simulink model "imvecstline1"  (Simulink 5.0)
settings: Solver=ode45  StartTime=0.0  StopTime=2.5  MaxStep=5e-4  RelTol=1e-3
libraries: simulink x1

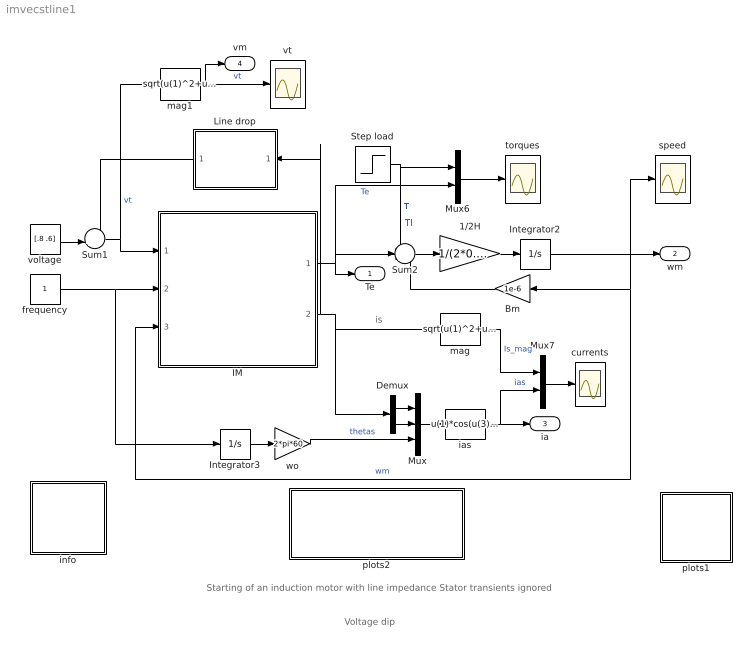
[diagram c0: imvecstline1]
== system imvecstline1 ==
  note: is
  note: Starting of an induction motor with line impedance Stator transients ignored
  note: Voltage dip
  note: Tl
  1/2H : Gain  Gain=1/(2*0.3)
  Bm : Gain  Orientation=left  Gain=1e-6
  Demux : Demux  Outputs=2
  IM : Subsystem  mask(Inductionmachine){Rs=0.01, Rr=0.02, Lsl=0.10, Lrl=0.10, Lm=4.50, wo=2*pi*60}
      mask prompts: Rs "Stator resistance [pu]"; Rr "Rotor resistance [pu]"; Lsl "Stator leakage inductance [pu]"; Lrl "Rotor leakage inductance [pu]"; Lm "Magnetizing inductance [pu]"; wo "Base frequency [rad/s]"
      mask help: Induction motor subsystem model using state space formulation in an arbitrary reference frame k. Parameters are expressed in per unit.
  Integrator2 : Integrator
  Integrator3 : Integrator
  Line drop : Subsystem  Orientation=left  mask{Rline=0.01, Lline=0.05, wo=2*pi*60}
      mask prompts: Rline "Rline [ pu]"; Lline "Lline [pu]"; wo "wo [rad/s]"
  Mux : Mux  Inputs=3
  Mux6 : Mux  Inputs=2
  Mux7 : Mux  Inputs=2
  Step load : Step  Time=2  Before=0.0  SampleTime=0
  Sum1 : Sum  Inputs=-+|
  Sum2 : Sum  Inputs=-+-
  currents : Scope
  frequency : Constant
  ias : Fcn  Expr=u(1)*cos(u(3))-u(2)*sin(u(3))
  info : Subsystem
  mag : Fcn  Expr=sqrt(u(1)^2+u(2)^2)
  mag1 : Fcn  Expr=sqrt(u(1)^2+u(2)^2)
  plots1 : Subsystem
  plots2 : Subsystem
  speed : Scope
  torques : Scope
  voltage : Constant  Value=[.8 .6]
  vt : Scope
  wo : Gain  Gain=2*pi*60
  Te : Outport
  wm : Outport  Port=2
  ia : Outport  Port=3
  vm : Outport  Port=4
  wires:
  frequency/1 -> Integrator3/1, IM/2(wk)
  Demux/1 -> Mux/1
  Demux/2 -> Mux/2
  mag/1 -> Mux7/1  "Is_mag"
  Sum2/1 -> 1/2H/1
  1/2H/1 -> Integrator2/1
  wo/1 -> Mux/3  "thetas"
  Bm/1 -> Sum2/3
  Integrator2/1 -> IM/3(wm), Bm/1, speed/1, wm/1  "wm"
  IM/1(Te) -> Sum2/2, Mux6/2, Te/1  "Te"
  IM/2(is) -> mag/1, Demux/1, Line drop/1(i_in)
  Mux6/1 -> torques/1
  Step load/1 -> Mux6/1, Sum2/1  "Tl"
  voltage/1 -> Sum1/2
  Line drop/1(v_out) -> Sum1/1
  Mux/1 -> ias/1
  Integrator3/1 -> wo/1
  Sum1/1 -> IM/1(vs), mag1/1  "vt"
  mag1/1 -> vt/1, vm/1  "vt"
  Mux7/1 -> currents/1
  ias/1 -> Mux7/2, ia/1  "ias"

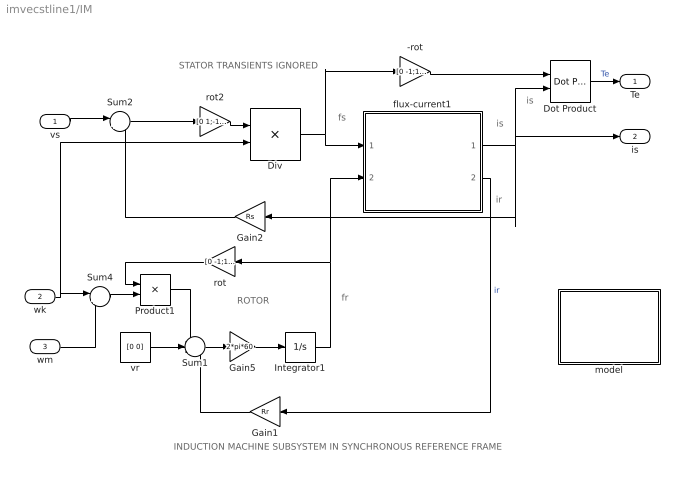
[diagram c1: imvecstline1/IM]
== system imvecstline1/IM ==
  note: ROTOR
  note: fs
  note: fr
  note: is
  note: is
  note: INDUCTION MACHINE SUBSYSTEM IN SYNCHRONOUS REFERENCE FRAME
  note: ir
  note: STATOR TRANSIENTS IGNORED
  vs : Inport
  wk : Inport  Port=2
  wm : Inport  Port=3
  -rot : Gain  Gain=[0 -1;1 0]  Multiplication=Matrix(K*u)
  Div : Product  Inputs=*/  Multiplication=Matrix(*)
  Dot Product : simulink/Math Operations/Dot Product
  Gain1 : Gain  Orientation=left  Gain=Rr
  Gain2 : Gain  Orientation=left  Gain=Rs
  Gain5 : Gain  Gain=2*pi*60
  Integrator1 : Integrator  InitialCondition=[0 0]
  Product1 : Product
  Sum1 : Sum  Inputs=-+-
  Sum2 : Sum  Inputs=|+-
  Sum4 : Sum  Inputs=|+-
  flux-current1 : Subsystem
  model : Subsystem
  rot : Gain  Orientation=left  Gain=[0 -1;1 0]  Multiplication=Matrix(K*u)
  rot2 : Gain  Gain=[0 1;-1 0]  Multiplication=Matrix(K*u)
  vr : Constant  Value=[0 0]
  Te : Outport
  is : Outport  Port=2
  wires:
  vr/1 -> Sum1/2
  Gain1/1 -> Sum1/3
  flux-current1/2(ir) -> Gain1/1  "ir"
  Integrator1/1 -> flux-current1/2(fr), rot/1
  Product1/1 -> Sum1/1
  rot/1 -> Product1/1
  Sum4/1 -> Product1/2
  Sum1/1 -> Gain5/1
  Gain5/1 -> Integrator1/1
  flux-current1/1(is) -> Dot Product/2, is/1, Gain2/1
  Dot Product/1 -> Te/1  "Te"
  wk/1 -> Sum4/1, Div/2
  wm/1 -> Sum4/2
  rot2/1 -> Div/1
  Div/1 -> flux-current1/1(fs), -rot/1
  -rot/1 -> Dot Product/1
  Sum2/1 -> rot2/1
  vs/1 -> Sum2/1
  Gain2/1 -> Sum2/2

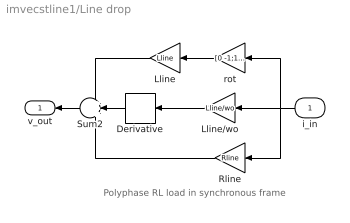
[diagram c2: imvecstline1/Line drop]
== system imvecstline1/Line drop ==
  note: Polyphase RL load in synchronous frame
  i_in : Inport  Orientation=left
  Derivative : Derivative  Orientation=left
  Lline : Gain  Orientation=left  Gain=Lline
  Lline/wo : Gain  Orientation=left  Gain=Lline/wo
  Rline : Gain  Orientation=left  Gain=Rline
  Sum2 : Sum  Orientation=left  Inputs=+++
  rot : Gain  Orientation=left  Gain=[0 -1;1 0]  Multiplication=Matrix(K*u)
  v_out : Outport  Orientation=left
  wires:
  Sum2/1 -> v_out/1
  Lline/wo/1 -> Derivative/1
  i_in/1 -> Lline/wo/1, rot/1, Rline/1
  rot/1 -> Lline/1
  Derivative/1 -> Sum2/2
  Lline/1 -> Sum2/1
  Rline/1 -> Sum2/3

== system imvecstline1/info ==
  note: Starting of an induction motor
  note: This demonstration illustrates the line starting of an induction motor at no load in the presence of a line impedance between the source and the motor.You will be able to observe the voltage dip associated with the high initial inrush current. To modify the machine parameters, double click the induction motor block. The model ignores the stator transients ( dfs/dt=0 ).

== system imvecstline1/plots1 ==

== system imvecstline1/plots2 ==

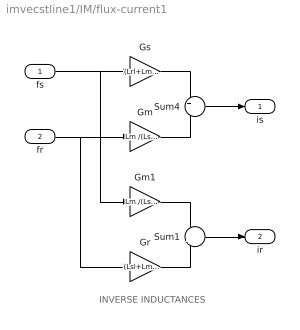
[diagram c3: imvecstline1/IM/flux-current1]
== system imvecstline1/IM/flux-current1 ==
  note: INVERSE INDUCTANCES
  fs : Inport
  fr : Inport  Port=2
  Gm : Gain  Gain=Lm /(Lsl*Lrl+Lsl*Lm+Lrl*Lm)
  Gm1 : Gain  Gain=Lm /(Lsl*Lrl+Lsl*Lm+Lrl*Lm)
  Gr : Gain  Gain=(Lsl+Lm )/(Lsl*Lrl+Lsl*Lm+Lrl*Lm)
  Gs : Gain  Gain=(Lrl+Lm) /(Lsl*Lrl+Lsl*Lm+Lrl*Lm)
  Sum1 : Sum  Inputs=-+
  Sum4 : Sum  Inputs=+-
  is : Outport
  ir : Outport  Port=2
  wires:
  fs/1 -> Gs/1, Gm1/1
  Gs/1 -> Sum4/1
  fr/1 -> Gm/1, Gr/1
  Gm/1 -> Sum4/2
  Sum4/1 -> is/1
  Gm1/1 -> Sum1/1
  Gr/1 -> Sum1/2
  Sum1/1 -> ir/1

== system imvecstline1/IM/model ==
  note: Mathematical model of the induction machine. State vector formulation in an arbitrary dq common reference frame. Per unit description.
  note: Electrical system equations: vs = Rs is + wk M(pi/2) fs (stator transients ignored) vr = Rr ir + 1/wo (dfr/dt) + (wk - wm) M(pi/2) fr where the variables i, v, and f are 2-dimensional space vectors; for instance is = [ids iqs] and so forth, wk is the speed of the reference frame, wm the rotor speed, and M(pi/2)represents a 90o space rotator namely M(pi/2) = [0 -1;1 0] The flux linkage current relations are: fs = Ls is + Lm ir or is = Gs fs -Gm fr fr = Lm is + Lr ir ir = -Gm fs + Gr fr Ls =Lm +Lsl ; Lr = Lm +Lrl Mechanical system equations: Te = 2H (dwm/dt ) + Bm wm + Tl where Te = fs (cross) is = M(pi/2) fs (dot) is = fds iqs - fqs ids = fs x is = M(pi/2) fs . is = ir x fr = Lm (ir x is) = Lm/Lr (fr x is) = 1/Lm' (fr x fs) Lm' =Lm c/(1-c) c = 1 - Lm^2/(Ls Lr)
